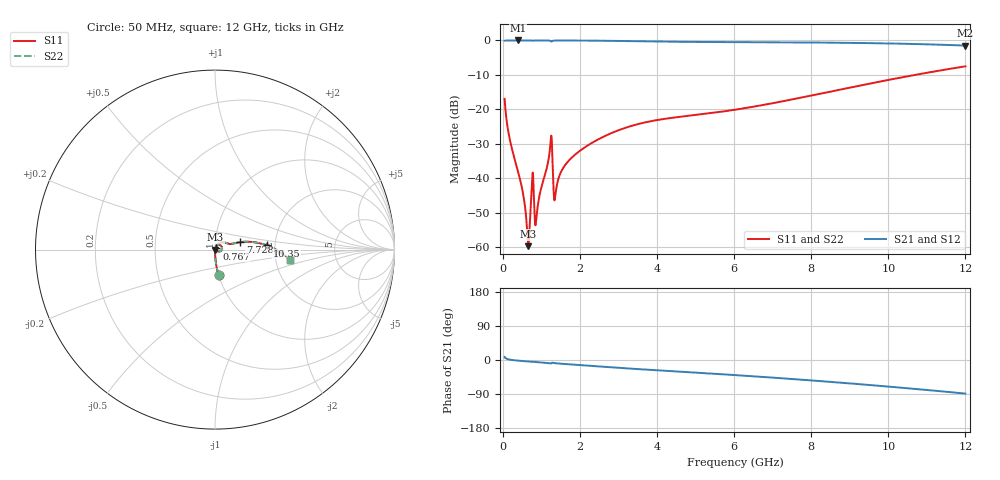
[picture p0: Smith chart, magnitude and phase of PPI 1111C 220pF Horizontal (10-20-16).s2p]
# MHz S MA R 50
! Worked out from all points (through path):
!   1601 points, 50 MHz to 12 GHz, reference 50 ohm
!   highest |S21| = -0.01 dB at 393.6 MHz (marker M1); lowest = -1.5 dB at 12 GHz (marker M2)
!   group delay of S21, straight-line fit = 20 ps
!   lowest |S11| = -59.8 dB at 662.4 MHz (marker M3), VSWR 1.00, Z = 50.1 - j0.0318 ohm
!   |S11| at or under -10 dB: start of sweep to 10.7 GHz
!   |S22| runs from -59.8 to -7.5 dB; largest |S21 - S12| = 0
!   S11 on the Smith chart (normalised r, x): 50 MHz: 1.00, -0.29; 767 MHz: 1.02, +0.01; 7.728 GHz: 1.32, +0.11; 10.35 GHz: 1.81, +0.09; 12 GHz: 2.40, -0.33
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50  0.1418 -82.0  0.9896 7.9  0.9896 7.9  0.1418 -82.0
184.4375  0.03647 -88.3  0.9989 1.0  0.9989 1.0  0.03647 -88.3
393.5625  0.01276 -88.8  0.9993 -1.6  0.9993 -1.6  0.01276 -88.8
520.5312  0.006286 -86.1  0.9992 -2.8  0.9992 -2.8  0.006286 -86.1
625.0938  0.002064 -68.4  0.9991 -3.7  0.9991 -3.7  0.002064 -68.4
662.4375  0.001028 -18.0  0.999 -4.0  0.999 -4.0  0.001028 -18.0
767  0.0101 38.0  0.9925 -5.0  0.9925 -5.0  0.0101 38.0
886.5  0.003069 55.8  0.9985 -5.5  0.9985 -5.5  0.003069 55.8
1230.062  0.02812 59.3  0.9891 -8.9  0.9891 -8.9  0.02812 59.3
1259.938  0.04152 21.2  0.9637 -8.8  0.9637 -8.8  0.04152 21.2
1342.094  0.004741 17.1  0.9956 -8.2  0.9956 -8.2  0.004741 17.1
1371.969  0.006004 50.5  0.9968 -8.5  0.9968 -8.5  0.006004 50.5
1581.094  0.01439 70.6  0.9975 -10.3  0.9975 -10.3  0.01439 70.6
2044.156  0.02595 67.1  0.9954 -13.7  0.9954 -13.7  0.02595 67.1
2962.812  0.04861 52.1  0.984 -20.3  0.984 -20.3  0.04861 52.1
4038.312  0.07025 32.7  0.9628 -27.4  0.9628 -27.4  0.07025 32.7
6025  0.09854 19.0  0.945 -39.8  0.945 -39.8  0.09854 19.0
7727.875  0.1473 16.4  0.9355 -51.8  0.9355 -51.8  0.1473 16.4
8019.156  0.1591 15.6  0.9331 -54.0  0.9331 -54.0  0.1591 15.6
10013.31  0.2676 6.6  0.9042 -70.3  0.9042 -70.3  0.2676 6.6
10349.41  0.2907 4.5  0.8964 -73.2  0.8964 -73.2  0.2907 4.5
12000  0.4208 -7.8  0.8417 -88.6  0.8417 -88.6  0.4208 -7.8
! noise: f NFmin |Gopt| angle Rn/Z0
50  0.0003689  0.865  0.3876  0.0005866
1372  0.006311  0.7927  8.231  0.006252
2701  0.01636  0.8404  16.09  0.0213
4031  0.03621  0.8917  23.81  0.06974
5360  0.04892  0.8961  31.3  0.09538
6682  0.05604  0.8911  38.45  0.0999
8012  0.062  0.8868  45.32  0.1014
9341  0.06809  0.8851  51.85  0.1041
1.067e+04  0.07475  0.8859  58.02  0.109
1.2e+04  0.0822  0.8889  63.84  0.1161
